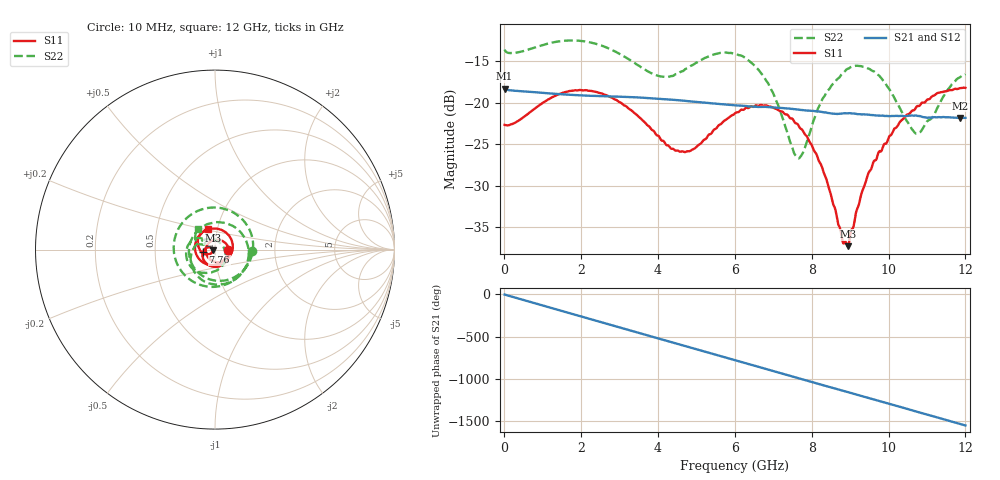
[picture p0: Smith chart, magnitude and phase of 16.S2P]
!Agilent Technologies,E5071C,MY46316741,A.11.02
!Date: Fri Apr 15 15:50:20 2022
!Data & Calibration Information:
!Freq	S11:SOLT2(ON)	S21:SOLT2(ON)	S12:SOLT2(ON)	S22:SOLT2(ON)
!PortZ  Port1:50+j0  Port2:50+j0
!Above PortZ is port z conversion or system Z0 setting when saving the data.
!When reading, reference impedance value at option line is always used.
# Hz S dB R 50
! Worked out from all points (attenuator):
!   1200 points, 10 MHz to 12 GHz, reference 50 ohm
!   highest |S21| = -18.33 dB at 10 MHz (marker M1); lowest = -21.9 dB at 11.87 GHz (marker M2)
!   lowest |S11| = -37.3 dB at 8.94 GHz (marker M3), VSWR 1.03, Z = 48.7 - j0.447 ohm
!   |S11| at or under -10 dB: start of sweep to end of sweep
!   |S22| runs from -26.7 to -12.5 dB; largest |S21 - S12| = 0.00072
!   S11 on the Smith chart (normalised r, x): 10 MHz: 1.16, -0.00; 7.76 GHz: 0.87, -0.02; 12 GHz: 0.91, +0.22
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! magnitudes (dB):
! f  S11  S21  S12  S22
! 10 MHz  -22.7  -18.3  -18.3  -13.6
! 1.38 GHz  -19.1  -19.0  -19.0  -12.7
! 2.01 GHz  -18.5  -19.1  -19.1  -12.6
! 2.98 GHz  -19.9  -19.3  -19.3  -14.1
! 4.01 GHz  -24.0  -19.5  -19.5  -16.8
! 4.4 GHz  -25.6  -19.7  -19.7  -16.8
! 4.82 GHz  -25.9  -19.8  -19.8  -15.7
! 5.47 GHz  -23.2  -20.1  -20.1  -14.2
! 6.01 GHz  -21.3  -20.3  -20.3  -14.2
! 6.77 GHz  -20.4  -20.5  -20.5  -17.0
! 7.09 GHz  -20.8  -20.6  -20.6  -19.9
! 7.56 GHz  -22.4  -20.8  -20.8  -26.2
! 7.76 GHz  -23.3  -20.9  -20.9  -26.1
! 8.01 GHz  -25.2  -21.0  -21.0  -22.7
! 8.35 GHz  -28.8  -21.2  -21.2  -19.1
! 8.8 GHz  -36.5  -21.3  -21.3  -16.5
! 8.94 GHz  -37.3  -21.3  -21.3  -15.9
! 9.46 GHz  -28.7  -21.4  -21.4  -15.9
! 10.01 GHz  -24.2  -21.6  -21.6  -18.3
! 10.75 GHz  -20.4  -21.6  -21.6  -23.7
! 11.87 GHz  -18.3  -21.9  -21.8  -16.9
! 12 GHz  -18.2  -21.8  -21.8  -16.6
